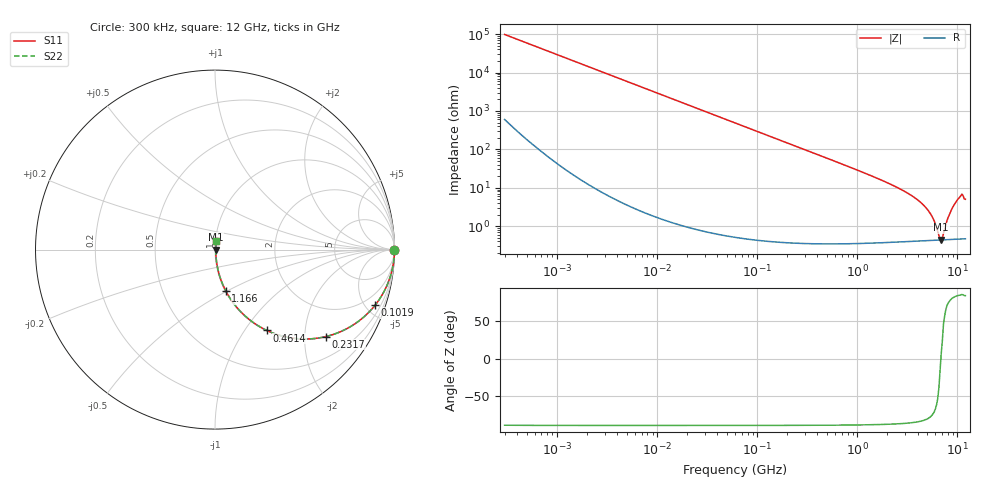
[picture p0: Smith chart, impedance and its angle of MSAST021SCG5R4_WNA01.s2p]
! MSAST021SCG5R4_WNA01  S-PARAMETER MODEL  ( General Type )
! Model Generated by TAIYO YUDEN Corporation (http://www.ty-top.com)
! Version 2.0
! TAIYO YUDEN Control No. 181101
! Copyright(c) 2015 TAIYO YUDEN CO.,LTD. All Rights Reserved.
! Product Description (link to TY-COMPAS)
! https://ds.yuden.co.jp/TYCOMPAS/or/detail?pn=MSAST021SCG5R4CWNA01&u=M
! Products Name : Multilayer Ceramic Capacitors
! Characteristics :
!  Capacitance : 5.4 pF , Rated Voltage : 25V , TCC : CG / C0G
!  Case Size : 0.25 x 0.125 / 0.0098 x 0.0049 [mm/inch] , Thickness : 0.125 / 0.0049 [mm/inch]
!  (Conditions: Temperature = 25 degC , DC Bias Current/Voltage = 0A / 0V)
! External Node Assignments :
!  1  o---| |---o  2
! GND o---------o GND
! Frequency Range : 0.3MHz  -  12000MHz  [ 401 STEP ]
# MHz S RI R 50
! Freq[MHz].  S11 Real  S11 Imag  S21 Real  S21 Imag  S12 Real  S12 Imag  S22 Real  S22 Imag
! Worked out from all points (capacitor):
!   401 points, 300 kHz to 12 GHz, reference 50 ohm
!   read as one part in series: C = 5.4 pF near 316.3 kHz
!   lowest |Z| = 442 mohm at 6.88 GHz (marker M1)
!   series resonance near 6.83 GHz, so ESL is about 100 pH
!   S11 on the Smith chart (normalised r, x): 300 kHz: open; 101.9 MHz: 1.01, -5.78; 231.7 MHz: 1.01, -2.54; 461.4 MHz: 1.01, -1.27; 1.166 GHz: 1.01, -0.49; 12 GHz: 1.01, +0.10
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0.3  1 -0.00102  7.26e-06 0.00102  7.26e-06 0.00102  1 -0.00102
1.769972  1 -0.00601  4.17e-05 0.00601  4.17e-05 0.00601  1 -0.00601
10.44266  0.9987 -0.0354  0.00127 0.0354  0.00127 0.0354  0.9987 -0.0354
27.82928  0.9911 -0.0936  0.0089 0.0936  0.0089 0.0936  0.9911 -0.0936
60  0.96 -0.1954  0.04 0.1954  0.04 0.1954  0.96 -0.1954
101.9188  0.8928 -0.3086  0.1072 0.3086  0.1072 0.3086  0.8928 -0.3086
231.6935  0.6172 -0.4847  0.3828 0.4847  0.3828 0.4847  0.6172 -0.4847
353.9943  0.4085 -0.4895  0.5915 0.4895  0.5915 0.4895  0.4085 -0.4895
461.3684  0.289 -0.4506  0.711 0.4506  0.711 0.4506  0.289 -0.4506
723.8279  0.1416 -0.3444  0.8584 0.3444  0.8584 0.3444  0.1416 -0.3444
1166.079  0.0597 -0.2298  0.9403 0.2298  0.9403 0.2298  0.0597 -0.2298
2088.533  0.0197 -0.1248  0.9803 0.1248  0.9803 0.1248  0.0197 -0.1248
3364.605  0.00829 -0.0653  0.9917 0.0653  0.9917 0.0653  0.00829 -0.0653
4623.766  0.00531 -0.0339  0.9947 0.0339  0.9947 0.0339  0.00531 -0.0339
5565.855  0.00456 -0.0173  0.9954 0.0173  0.9954 0.0173  0.00456 -0.0173
6524.734  0.00436 -0.00354  0.9956 0.00354  0.9956 0.00354  0.00436 -0.00354
6879.757  0.00437 0.000478  0.9956 -0.000478  0.9956 -0.000478  0.00437 0.000478
7254.098  0.00442 0.00469  0.9956 -0.00469  0.9956 -0.00469  0.00442 0.00469
8281.503  0.00483 0.0188  0.9952 -0.0188  0.9952 -0.0188  0.00483 0.0188
9454.42  0.00603 0.0384  0.994 -0.0384  0.994 -0.0384  0.00603 0.0384
10793.46  0.00839 0.0612  0.9916 -0.0612  0.9916 -0.0612  0.00839 0.0612
12000  0.00712 0.0493  0.9929 -0.0493  0.9929 -0.0493  0.00712 0.0493
